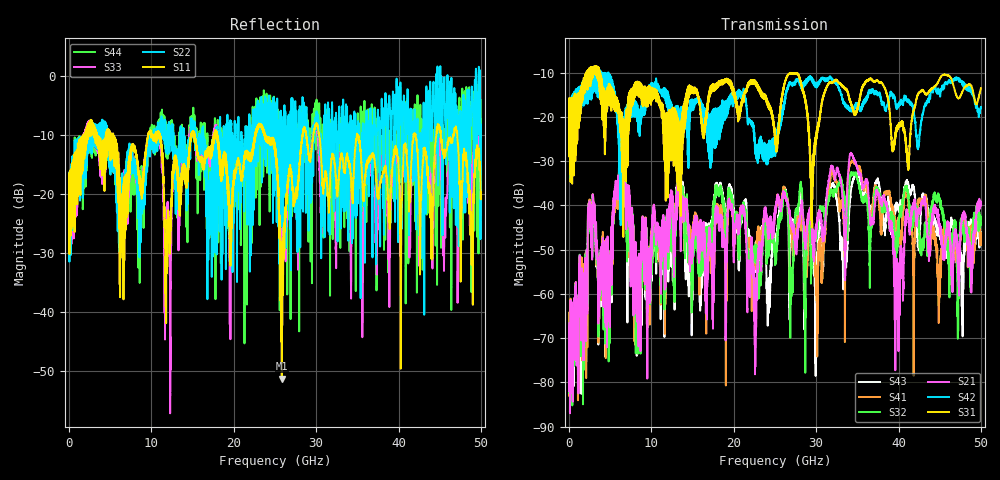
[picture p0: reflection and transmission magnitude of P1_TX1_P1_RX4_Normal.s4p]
!Keysight Technologies,N5225B,MY57041031,A.13.20.10
!Date: Friday, May 31, 2019 11:18:47
!Correction: S11(Full 4 Port(1,2,3,4))
!S12(Full 4 Port(1,2,3,4))
!S13(Full 4 Port(1,2,3,4))
!S14(Full 4 Port(1,2,3,4))
!S21(Full 4 Port(1,2,3,4))
!S22(Full 4 Port(1,2,3,4))
!S23(Full 4 Port(1,2,3,4))
!S24(Full 4 Port(1,2,3,4))
!S31(Full 4 Port(1,2,3,4))
!S32(Full 4 Port(1,2,3,4))
!S33(Full 4 Port(1,2,3,4))
!S34(Full 4 Port(1,2,3,4))
!S41(Full 4 Port(1,2,3,4))
!S42(Full 4 Port(1,2,3,4))
!S43(Full 4 Port(1,2,3,4))
!S44(Full 4 Port(1,2,3,4))
!S4P File: Measurements: <S11,S12,S13,S14>,
!<S21,S22,S23,S24>,
!<S31,S32,S33,S34>,
!<S41,S42,S43,S44>:
# Hz S  dB  R 50.0
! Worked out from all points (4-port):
!   5000 points, 10 MHz to 50 GHz, reference 50 ohm
!   strongest paths, dB at 10 MHz, 12.51 GHz, 25.01 GHz, 37.51 GHz, 50 GHz:
!     S31: -19.5, -29.3, -24.6, -11.8, -13.5
!     S42: -19.4, -19.4, -25.8, -14.9, -17.7
!     S21: -66.7, -38.1, -42.4, -37.6, -39.2
!     S32: -67.1, -41.9, -53.5, -36.5, -44.0
!     S41: -64.2, -38.8, -42.8, -37.5, -48.9
!     S43: -70.1, -43.2, -49.1, -34.2, -46.0
!   lowest |S11| = -51.3 dB at 25.83 GHz (marker M1), VSWR 1.01, Z = 50 + j0.27 ohm
!   |S11| at or under -10 dB: 18.01 GHz to 22.61 GHz (4.596 GHz wide, 22.6 % of centre); 30.38 GHz to 34.94 GHz (4.563 GHz wide, 14 % of centre); 34.98 GHz to 41.82 GHz (6.842 GHz wide, 17.8 % of centre)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
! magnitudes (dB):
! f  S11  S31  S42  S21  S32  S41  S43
! 10 MHz  -19.9  -19.5  -19.4  -66.7  -67.1  -64.2  -70.1
! 6.4 GHz  -24.6  -23.1  -24.1  -29.1  -29.4  -29.9  -30.5
! 8.45 GHz  -16.8  -12.2  -19.1  -56.9  -55.0  -65.7  -61.9
! 13.34 GHz  -20.0  -24.2  -20.7  -34.5  -32.7  -34.1  -32.4
! 23.26 GHz  -8.2  -14.6  -26.0  -52.1  -55.5  -48.4  -47.8
! 25.83 GHz  -51.3  -16.0  -19.3  -39.5  -42.2  -38.5  -40.6
! 50 GHz  -19.7  -13.5  -17.7  -39.2  -44.0  -48.9  -46.0
